TYPE STR_AI :
STRUCT
VG101_Pressure	,
VG102_Pressure	,
//VG103_Pressure	,
VG104_Pressure	,
BA1_Pressure	,
MFC1_Flow	,
APC_Temp	,	//TC01
Gate_Valve_Temp	,		//TC13
Gate_Valve_Temp_Monitor,	//TC14
//IGS_Temp1	,	//TC35
//IGS_Temp2	,	//TC36
//IGS_Temp3	,	//TC35
//IGS_Temp4	,	//TC36
Lid_Temp	,	//TC02
//Lid_Temp_Monitor1	,	//TC03
//Lid_Temp_Monitor2	,	//TC04
//Tape_Temp1	,	//TC31
//Tape_Temp2	,	//TC32
AV102_Temp	,
AV101_Temp	,
AV104_Temp	,
AV105_Temp	,
//BA01_Temp	,
//VG103_Pipe_Temp	,
Exhaust1_3_Temp	,
Exhaust4_7_Temp	,
VG101_Pipe_Temp	,
Chamber_Temp1	,	//TC05
Chamber_Temp2	,	//TC06
Chamber_Temp3	,	//TC07
//Chamber_Temp_Monitor,	//TC12
Stage_Temp1	,		//TC08
Stage_Temp1_Monitor	,
Stage_Temp2	,		//TC09
Stage_Temp2_Monitor	,
Stage_Temp3	,		//TC10
Stage_Temp3_Monitor	,
Stage_Temp4	,
Stage_Temp4_Monitor	:REAL;		//TC11	

PG_PS1_Value	,
//PG_PS2_Value	,
//PG_PS3_Value	,
//PG_PS4_Value	,
//PG_PS5_Value	,
//PG_PS6_Value	,
//PG_PS7_Value	,
//PG_PS8_Value	,
//PG_PS9_Value	,
PS1_Value	,
//PS2_Value	,
MS1_Value	:REAL;
//GD01_Value	,
//GD02_Value	:REAL;

APC:VAT_IN;

TMP:TMP_IN;

Water_Flow:REAL;

END_STRUCT
END_TYPE
